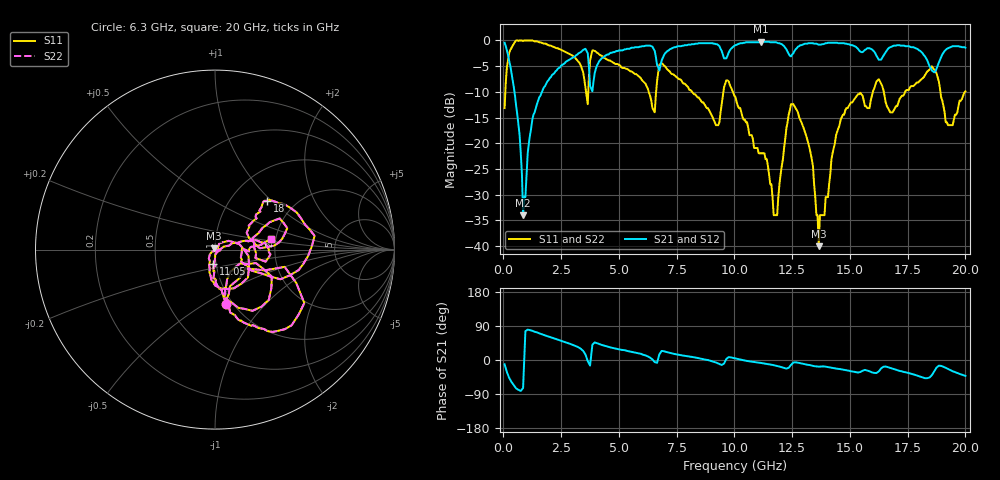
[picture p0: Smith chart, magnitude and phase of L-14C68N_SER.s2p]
# MHZ S MA R 50
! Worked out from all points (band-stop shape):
!   400 points, 50 MHz to 20 GHz, reference 50 ohm
!   highest |S21| = -0.26 dB at 11.15 GHz (marker M1); lowest = -34.0 dB at 850 MHz (marker M2)
!   |S21| within 3 dB of the highest: 6.909 GHz to 9.536 GHz (2.627 GHz wide, 32 % of centre); 9.671 GHz to 16.19 GHz (6.517 GHz wide, 50.4 % of centre)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
!   lowest |S11| = -40.0 dB at 13.65 GHz (marker M3), VSWR 1.02, Z = 49.3 + j0.719 ohm
!   |S11| at or under -10 dB: 8.169 GHz to 9.523 GHz (1.354 GHz wide, 15.3 % of centre); 9.934 GHz to 15.99 GHz (6.06 GHz wide, 46.7 % of centre); 18.92 GHz to 19.98 GHz (1.063 GHz wide, 5.46 % of centre)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
!   |S22| runs from -40.0 to 0.0 dB; largest |S21 - S12| = 0
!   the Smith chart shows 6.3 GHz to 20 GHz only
!   S11 on the Smith chart (normalised r, x): 6.3 GHz: 0.93, -0.62; 11.05 GHz: 0.97, -0.15; 18 GHz: 1.46, +0.95; 20 GHz: 1.90, +0.24
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50  0.22 71.0  0.95 -11.3  0.95 -11.3  0.22 71.0
700  1 11.0  0.12 -80.2  0.12 -80.2  1 11.0
850  0.99 5.0  0.02 -73.9  0.02 -73.9  0.99 5.0
1550  0.96 -15.2  0.28 70.3  0.28 70.3  0.96 -15.2
3400  0.53 -60.6  0.79 26.8  0.79 26.8  0.53 -60.6
3650  0.24 -13.5  0.75 -3.1  0.75 -3.1  0.24 -13.5
3850  0.8 -25.2  0.32 40.5  0.32 40.5  0.8 -25.2
6300  0.31 -78.5  0.89 7.9  0.89 7.9  0.31 -78.5
6700  0.49 -22.4  0.55 3.8  0.55 3.8  0.49 -22.4
10050  0.28 -79.5  0.9 3.8  0.9 3.8  0.28 -79.5
11050  0.08 -97.9  0.96 -6.8  0.96 -6.8  0.08 -97.9
11150  0.08 -92.5  0.97 -7.8  0.97 -7.8  0.08 -92.5
11700  0.02 -71.9  0.96 -13.7  0.96 -13.7  0.02 -71.9
12450  0.24 -39.9  0.7 -13.0  0.7 -13.0  0.24 -39.9
13350  0.07 -114.1  0.94 -14.8  0.94 -14.8  0.07 -114.1
13650  0.01 133.2  0.91 -17.7  0.91 -17.7  0.01 133.2
14800  0.21 13.8  0.93 -26.6  0.93 -26.6  0.21 13.8
16700  0.21 14.8  0.85 -19.9  0.85 -19.9  0.21 14.8
18000  0.4 43.1  0.8 -42.9  0.8 -42.9  0.4 43.1
18850  0.4 -24.4  0.61 -15.1  0.61 -15.1  0.4 -24.4
19250  0.15 -16.6  0.84 -23.9  0.84 -23.9  0.15 -16.6
20000  0.32 10.4  0.85 -42.0  0.85 -42.0  0.32 10.4
